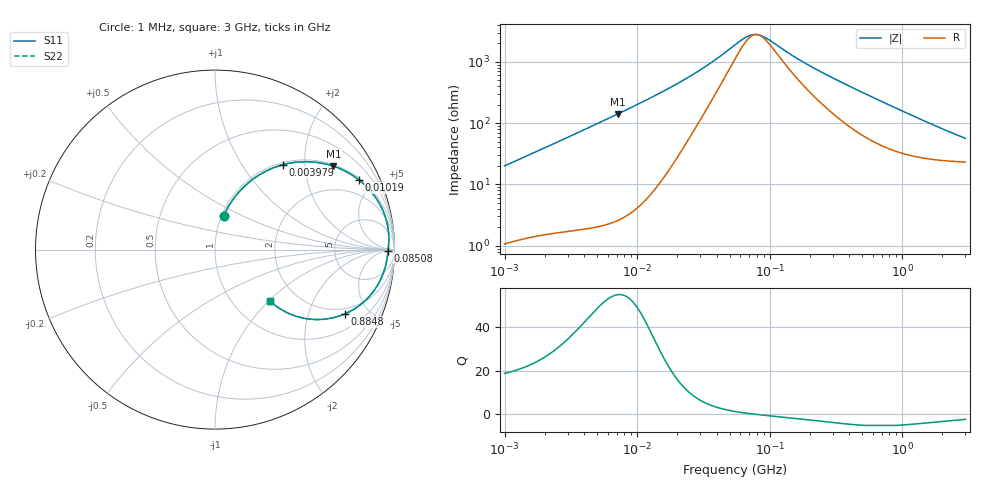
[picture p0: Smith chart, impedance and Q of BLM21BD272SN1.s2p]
! BLM21BD272SN1
# Hz S RI R 50
!Freq.(Hz) S11(Real) S11(Imag) S21(Real) S21(Imag) S12(Real) S12(Imag) S22(Real) S22(Imag)
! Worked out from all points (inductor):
!   401 points, 1 MHz to 3 GHz, reference 50 ohm
!   read as one part in series: L = 3.16 uH near 1.041 MHz
!   highest Q = 54.6 at 7.11 MHz (marker M1), where L = 3.14 uH
!   self-resonance near 80.32 MHz
!   S11 on the Smith chart (normalised r, x): 1 MHz: 1.02, +0.40; 3.979 MHz: 1.04, +1.56; 10.19 MHz: 1.09, +4.09; 85.08 MHz: 54, -9; 884.8 MHz: 1.70, -3.49; 3 GHz: 1.46, -1.03
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1000000  0.0479 0.1885  0.9521 -0.1885  0.9521 -0.1885  0.0479 0.1885
2055611  0.1495 0.3382  0.8505 -0.3382  0.8505 -0.3382  0.1495 0.3382
2775447  0.2347 0.4087  0.7653 -0.4087  0.7653 -0.4087  0.2347 0.4087
3823119  0.3616 0.4684  0.6384 -0.4684  0.6384 -0.4684  0.3616 0.4684
3979270  0.3797 0.4736  0.6203 -0.4736  0.6203 -0.4736  0.3797 0.4736
5372736  0.5253 0.4895  0.4747 -0.4895  0.4747 -0.4895  0.5253 0.4895
7110411  0.6602 0.4646  0.3398 -0.4646  0.3398 -0.4646  0.6602 0.4646
1.019448e7  0.8021 0.3882  0.1979 -0.3882  0.1979 -0.3882  0.8021 0.3882
1.461624e7  0.8941 0.2914  0.1059 -0.2914  0.1059 -0.2914  0.8941 0.2914
2.944989e7  0.9625 0.1297  0.0375 -0.1297  0.0375 -0.1297  0.9625 0.1297
5.477226e7  0.968 0.0401  0.032 -0.0401  0.032 -0.0401  0.968 0.0401
7.105049e7  0.9663 0.0122  0.0337 -0.0122  0.0337 -0.0122  0.9663 0.0122
8.507507e7  0.9647 -0.00566  0.0353 0.00566  0.0353 0.00566  0.9647 -0.00566
9.787053e7  0.9632 -0.0194  0.0368 0.0194  0.0368 0.0194  0.9632 -0.0194
1.49005e8  0.9566 -0.0625  0.0434 0.0625  0.0434 0.0625  0.9566 -0.0625
2.094008e8  0.9468 -0.1037  0.0532 0.1037  0.0532 0.1037  0.9468 -0.1037
4.480278e8  0.8849 -0.2302  0.1151 0.2302  0.1151 0.2302  0.8849 -0.2302
8.005644e8  0.7553 -0.343  0.2447 0.343  0.2447 0.343  0.7553 -0.343
8.848309e8  0.7231 -0.3585  0.2769 0.3585  0.2769 0.3585  0.7231 -0.3585
1.54974e9  0.5117 -0.3853  0.4883 0.3853  0.4883 0.3853  0.5117 -0.3853
2.221924e9  0.3862 -0.3435  0.6138 0.3435  0.6138 0.3435  0.3862 -0.3435
3e9  0.3085 -0.2887  0.6915 0.2887  0.6915 0.2887  0.3085 -0.2887
